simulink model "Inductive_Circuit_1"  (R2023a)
settings: Solver=VariableStepAuto  StartTime=0.0  StopTime=10.0  RelTol=1e-3
libraries: fl_lib x9

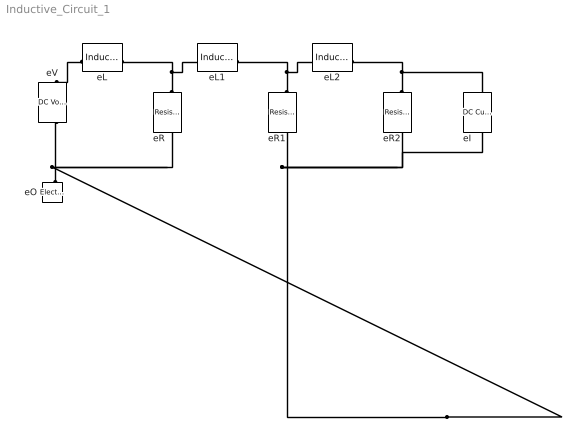
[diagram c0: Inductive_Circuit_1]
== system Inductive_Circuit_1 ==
  eI : fl_lib/Electrical/Electrical Sources/DC Current Source  i0=1 A
  eL : fl_lib/Electrical/Electrical Elements/Inductor  l=1e-6 H  r=0 Ohm  g=1e-9 1/Ohm  i_specify=off  i_priority=None  i=0 A  i_nominal_specify=off  i_nominal_unit=A  i_nominal_value=1  v_specify=off  v_priority=None  v=0 V  v_nominal_specify=off  v_nominal_unit=V  v_nominal_value=1  i_L_specify=off  i_L_priority=High  i_L=0 A  i_L_nominal_specify=off  i_L_nominal_unit=A  i_L_nominal_value=1
  eL1 : fl_lib/Electrical/Electrical Elements/Inductor  l=1e-6 H  r=0 Ohm  g=1e-9 1/Ohm  i_specify=off  i_priority=None  i=0 A  i_nominal_specify=off  i_nominal_unit=A  i_nominal_value=1  v_specify=off  v_priority=None  v=0 V  v_nominal_specify=off  v_nominal_unit=V  v_nominal_value=1  i_L_specify=off  i_L_priority=High  i_L=0 A  i_L_nominal_specify=off  i_L_nominal_unit=A  i_L_nominal_value=1
  eL2 : fl_lib/Electrical/Electrical Elements/Inductor  l=1e-6 H  r=0 Ohm  g=1e-9 1/Ohm  i_specify=off  i_priority=None  i=0 A  i_nominal_specify=off  i_nominal_unit=A  i_nominal_value=1  v_specify=off  v_priority=None  v=0 V  v_nominal_specify=off  v_nominal_unit=V  v_nominal_value=1  i_L_specify=off  i_L_priority=High  i_L=0 A  i_L_nominal_specify=off  i_L_nominal_unit=A  i_L_nominal_value=1
  eO : fl_lib/Electrical/Electrical Elements/Electrical Reference
  eR : fl_lib/Electrical/Electrical Elements/Resistor  R=1 Ohm  i_specify=off  i_priority=None  i=0 A  i_nominal_specify=off  i_nominal_unit=A  i_nominal_value=1  v_specify=off  v_priority=None  v=0 V  v_nominal_specify=off  v_nominal_unit=V  v_nominal_value=1
  eR1 : fl_lib/Electrical/Electrical Elements/Resistor  R=1 Ohm  i_specify=off  i_priority=None  i=0 A  i_nominal_specify=off  i_nominal_unit=A  i_nominal_value=1  v_specify=off  v_priority=None  v=0 V  v_nominal_specify=off  v_nominal_unit=V  v_nominal_value=1
  eR2 : fl_lib/Electrical/Electrical Elements/Resistor  R=1 Ohm  i_specify=off  i_priority=None  i=0 A  i_nominal_specify=off  i_nominal_unit=A  i_nominal_value=1  v_specify=off  v_priority=None  v=0 V  v_nominal_specify=off  v_nominal_unit=V  v_nominal_value=1
  eV : fl_lib/Electrical/Electrical Sources/DC Voltage Source  v0=1 V
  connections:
  eO/LConn1 -- eR/RConn1 -- eI/RConn1 -- eR2/RConn1 -- eR1/RConn1 -- eV/RConn1
  eL/LConn1 -- eV/LConn1
  eR/LConn1 -- eL1/LConn1 -- eL/RConn1
  eR1/LConn1 -- eL1/RConn1 -- eL2/LConn1
  eR2/LConn1 -- eI/LConn1 -- eL2/RConn1
